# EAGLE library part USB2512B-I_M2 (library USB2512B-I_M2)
Microchip USB2512B-I/M2, USB Controller, USB 2.0, 3.3 V, 36-Pin SQFN Source: Datasheet
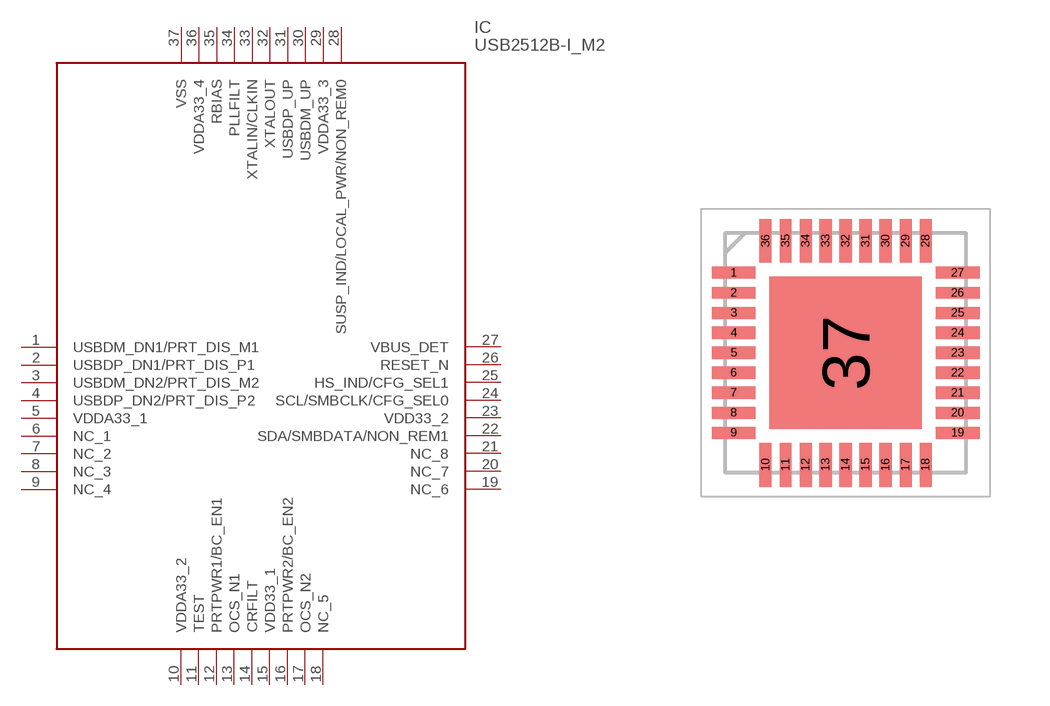
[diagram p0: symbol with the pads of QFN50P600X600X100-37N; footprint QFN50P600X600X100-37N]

Designator prefix IC

## USB2512B-I_M2 (Arrow_Part_Number: USB2512B-I/M2; Arrow_Price-Stock: https://www.arrow.com/en/products/usb2512b-im2/microchip-technology?region=nac; Description: Microchip USB2512B-I/M2, USB Controller, USB 2.0, 3.3 V, 36-Pin SQFN; Height: 1mm; Manufacturer_Name: Microchip; Manufacturer_Part_Number: USB2512B-I/M2; Mouser_Part_Number: 579-USB2512B-I/M2; Mouser_Price-Stock: https://www.mouser.co.uk/ProductDetail/Microchip-Technology/USB2512B-I-M2?qs=uus7iwvxYD8%2FmTpAijPQAQ%3D%3D)  [QFN50P600X600X100-37N]
1  USBDM_DN1/PRT_DIS_M1
2  USBDP_DN1/PRT_DIS_P1
3  USBDM_DN2/PRT_DIS_M2
4  USBDP_DN2/PRT_DIS_P2
5  VDDA33_1
6  NC_1
7  NC_2
8  NC_3
9  NC_4
10  VDDA33_2
11  TEST
12  PRTPWR1/BC_EN1
13  OCS_N1
14  CRFILT
15  VDD33_1
16  PRTPWR2/BC_EN2
17  OCS_N2
18  NC_5
19  NC_6
20  NC_7
21  NC_8
22  SDA/SMBDATA/NON_REM1
23  VDD33_2
24  SCL/SMBCLK/CFG_SEL0
25  HS_IND/CFG_SEL1
26  RESET_N
27  VBUS_DET
28  SUSP_IND/LOCAL_PWR/NON_REM0
29  VDDA33_3
30  USBDM_UP
31  USBDP_UP
32  XTALOUT
33  XTALIN/CLKIN
34  PLLFILT
35  RBIAS
36  VDDA33_4
37  VSS

## Footprint QFN50P600X600X100-37N (pad centres in mm)
36-PIN SQFN
smd 1.1 x 0.3: 1 -2.8,2; 2 -2.8,1.5; 3 -2.8,1; 4 -2.8,0.5; 5 -2.8,0; 6 -2.8,-0.5; 7 -2.8,-1; 8 -2.8,-1.5; 9 -2.8,-2; 19 2.8,-2; 20 2.8,-1.5; 21 2.8,-1; 22 2.8,-0.5; 23 2.8,0; 24 2.8,0.5; 25 2.8,1; 26 2.8,1.5; 27 2.8,2
smd 0.3 x 1.1: 10 -2,-2.8; 11 -1.5,-2.8; 12 -1,-2.8; 13 -0.5,-2.8; 14 0,-2.8; 15 0.5,-2.8; 16 1,-2.8; 17 1.5,-2.8; 18 2,-2.8; 28 2,2.8; 29 1.5,2.8; 30 1,2.8; 31 0.5,2.8; 32 0,2.8; 33 -0.5,2.8; 34 -1,2.8; 35 -1.5,2.8; 36 -2,2.8
smd 3.8 x 3.8: 37 0,0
